(*
	Feekback1_UDINT/Feekback2_DINT 需要链接硬件
	bExecute上电延时再触发，NC server 准备好才能触发读取 脉冲当量
*)
FUNCTION_BLOCK FB_MutliTurnsEncoderCount
VAR_INPUT
	bExecute							:	BOOL;
	refAxis								:	REFERENCE TO axis_ref;
	eDataTpye							:	(eUDINT,eDINT)INT;
END_VAR
VAR
	Feekback1_UDINT		AT%I*			:	UDINT;
	Feekback2_DINT		AT%I*			:	DINT;
	
	Feekback_DINT 						:	DINT;
	Feekback_LINT						:	LINT;
	fbAdsReadScalingFactorNumerator		:	ADSREAD;
	fbAdsReadScalingFactorDenominator	:	ADSREAD;
	DeltaFeedback						:	LINT;
	fbSetPosition						:	MC_SetPosition;
	rtExecute							:	R_TRIG;
	eState								:	(eIDLE,eREAD_SCALINT_FACTOR,eCALCULATE,eSET_POSITION,eRECORD) := eIDLE;
END_VAR
VAR_OUTPUT
	Numerator							:	LREAL;
	Denominator							:	LREAL;
	SetPosition							:	LREAL;
	sLog								:	STRING(1023);
	bBusy								:	BOOL;
	bError								:	BOOL;
END_VAR
VAR PERSISTENT
	LastActPos							:	LREAL;
	LastFeedback						:	LINT;
END_VAR
VAR CONSTANT
	cNumerator							:	UDINT := 16#23;
	cDenominator						:	UDINT := 16#24;
END_VAR


// 数据输入
CASE eDataTpye OF 
	eUDINT :
			Feekback_DINT := TO_DINT(Feekback1_UDINT);
			Feekback_LINT := TO_LINT(Feekback_DINT);
	eDINT :
			Feekback_LINT := TO_LINT(Feekback2_DINT);	
END_CASE
rtExecute(CLK:= bExecute, Q=> );
CASE eState OF 
	eIDLE :
				IF rtExecute.Q THEN 
					IF NOT __ISVALIDREF(refAxis) THEN 
						sLog := 'Input data <refAxis> is not valid';
						bError := TRUE;
						RETURN;
					END_IF
					eState := eREAD_SCALINT_FACTOR;
					bBusy := TRUE;
					bError := FALSE;
					sLog := '';
					fbAdsReadScalingFactorNumerator(READ:= FALSE);
					fbAdsReadScalingFactorDenominator(READ:= FALSE);
					fbSetPosition(Axis:= refAxis,Execute:= FALSE);
				END_IF
	eREAD_SCALINT_FACTOR:
			fbAdsReadScalingFactorNumerator(
				NETID:= , 
				PORT:= 501, 
				IDXGRP:= 16#5000+refAxis.NcToPlc.AxisId, 
				IDXOFFS:= cNumerator, 
				LEN:= 8, 
				DESTADDR:= ADR(Numerator), 
				READ:= TRUE, 
				TMOUT:= , 
				BUSY=> , 
				ERR=> , 
				ERRID=> );
			fbAdsReadScalingFactorDenominator(
				NETID:= , 
				PORT:= 501, 
				IDXGRP:= 16#5000+refAxis.NcToPlc.AxisId, 
				IDXOFFS:= cDenominator, 
				LEN:= 8, 
				DESTADDR:= ADR(Denominator), 
				READ:= TRUE, 
				TMOUT:= , 
				BUSY=> , 
				ERR=> , 
				ERRID=> );
			IF fbAdsReadScalingFactorNumerator.ERR THEN 
				bBusy := FALSE;
				bError := TRUE;
				sLog := CONCAT(sLog,'fbAdsReadScalingFactorNumerator|');
				sLog := CONCAT(sLog,TO_STRING(fbAdsReadScalingFactorNumerator.ERRID));
				eState := eIdle;
			END_IF
			IF fbAdsReadScalingFactorDenominator.ERR THEN 
				bBusy := FALSE;
				bError := TRUE;
				sLog := CONCAT(sLog,'fbAdsReadScalingFactorDenominator|');
				sLog := CONCAT(sLog,TO_STRING(fbAdsReadScalingFactorDenominator.ERRID));
				eState := eIdle;
			END_IF
			
			IF NOT fbAdsReadScalingFactorNumerator.BUSY AND NOT fbAdsReadScalingFactorNumerator.ERR 
			AND NOT fbAdsReadScalingFactorDenominator.BUSY AND NOT fbAdsReadScalingFactorDenominator.ERR 
			THEN 
				fbAdsReadScalingFactorNumerator(READ:= FALSE);
				fbAdsReadScalingFactorDenominator(READ:= FALSE);
				eState := eCALCULATE;
			END_IF
	eCALCULATE :(* DeltaFeedback 结果最大 33位(*32位数据+1位符号*)，后面转64bit浮点数不丢数据*)
				DeltaFeedback := Feekback_LINT - LastFeedback; 
				IF DeltaFeedback > 16#8000_0000(*16#1_0000_0000/2*) THEN 
					DeltaFeedback := DeltaFeedback - 16#1_0000_0000;
				ELSIF DeltaFeedback < ((-1) * 16#8000_0000)(*16#1_0000_0000/2*) THEN 
					DeltaFeedback := DeltaFeedback + 16#1_0000_0000;
				END_IF
				SetPosition := LastActPos + TO_LREAL(DeltaFeedback) * Numerator / Denominator;
				eState := eSET_POSITION;
	eSET_POSITION:
				fbSetPosition.Options.ClearPositionLag := TRUE;// 清除跟随误差
				fbSetPosition(
					Axis:= refAxis, 
					Execute:= TRUE, 
					Position:= SetPosition, 
					Mode:= , (* RELATIVE=True, ABSOLUTE=False (Default) *)
					Options:= , 
					Done=> , 
					Busy=> , 
					Error=> , 
					ErrorID=> );
				IF fbSetPosition.Done THEN 
					eState := eRECORD;
					bBusy := FALSE;
					fbSetPosition(Axis:= refAxis,Execute:= FALSE);
				ELSIF fbSetPosition.Error THEN
					bBusy := FALSE;
					bError := TRUE;
					sLog := CONCAT(sLog,'fbSetPosition|');
					sLog := CONCAT(sLog,TO_STRING(fbSetPosition.ErrorID));
					eState := eIDLE;
				END_IF
	eRECORD :
				LastActPos := refAxis.NcToPlc.ActPos;
				LastFeedback := Feekback_LINT;
END_CASE

END_FUNCTION_BLOCK
